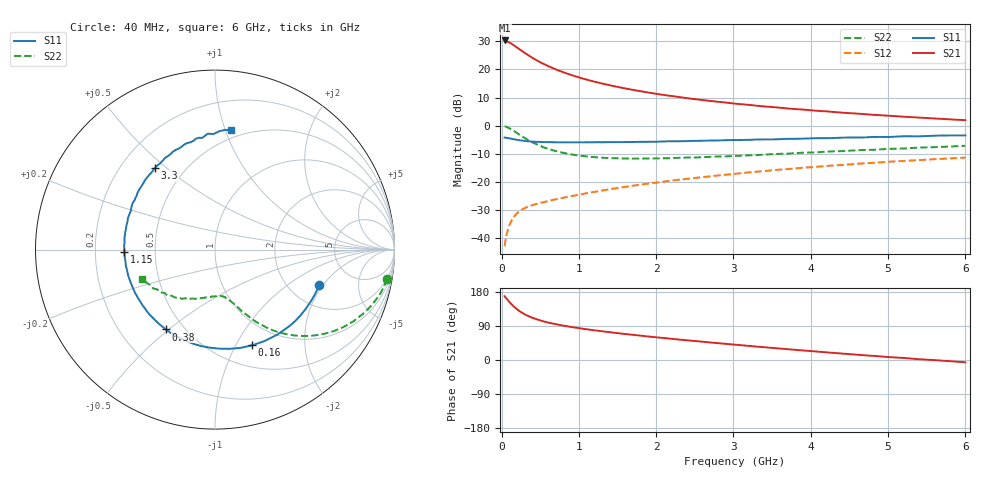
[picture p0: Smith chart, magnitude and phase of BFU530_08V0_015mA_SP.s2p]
! Filename:  P:\Prog\Test\Noise\ATS_data\Testdata_Net\03 Spar\BFU530_APG2013_40_A05_08p0V_015mA_SP_CM01_D.s2p
! Date/Time: Fri 26/Apr/2013 13:03:13
! BFU530_APG2013_40_A05_08p0V_1to25mA_SP_CM01_Bias6_R.s2p
! MDIF S-parameter v. bias file
! BFU530_APG2013_40_A05_08p0V_1to25mA_SP_CM01
! Date/time Wed Apr 24 16:58:28 2013
! VAR V_out= 8.0000
! VAR I_out= 14.9950
! VAR V_in= 0.8199
! VAR I_in= 0.1591
! Device data file deembeded for feedlines and parallel
! Original file: \03 Spar\BFU530_APG2013_40_A05_08p0V_015mA_SP_CM01_R.s2p
! Feed-files: PR047V01_250413_Feed1.s2p, PR047V01_250413_Feed2.s2p
! Parallel-file: PR047V01_250413_Par.s2p
# MHz S MA R 50
!  Freq-MHz  S11-mag  S11-arg  S21-mag  S21-arg  S12-mag  S12-arg  S22-mag  S22-arg
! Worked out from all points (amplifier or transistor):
!   98 points, 40 MHz to 6 GHz, reference 50 ohm
!   highest |S21| = 30.3 dB at 40 MHz (marker M1)
!   |S21| within 3 dB of that: start of sweep to 226.2 MHz
!   unconditionally stable (mu >= 1): 1.53 GHz to 3.802 GHz
!   at 300 MHz: K = 0.39, MSG = 27.6 dB, |S12| = -29.4 dB
!   at 1.6 GHz: K = 1.01, MAG = 16.8 dB, |S12| = -21.8 dB
!   at 6 GHz: K = 0.87, MSG = 6.7 dB, |S12| = -11.4 dB
!   S11 on the Smith chart (normalised r, x): 40 MHz: 2.89, -1.84; 160 MHz: 0.74, -1.17; 380 MHz: 0.40, -0.49; 1.15 GHz: 0.33, -0.01; 3.3 GHz: 0.34, +0.46; 6 GHz: 0.44, +1.05
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40  0.6132 -18.9  32.73 168.4  0.007166 82.0  0.9714 -9.7
50  0.6104 -23.6  32.58 165.4  0.008843 79.9  0.9648 -12.2
100  0.5949 -45.7  30.09 153.6  0.01661 71.2  0.8991 -23.4
120  0.5872 -54.0  29.08 149.0  0.01925 68.1  0.8681 -27.4
160  0.572 -68.8  26.75 141.0  0.02385 62.8  0.8031 -34.4
220  0.5524 -87.7  23.5 130.9  0.02904 57.2  0.708 -42.8
260  0.5432 -98.1  21.48 125.4  0.03172 54.5  0.6519 -47.2
320  0.5309 -111.1  18.88 118.5  0.03497 51.8  0.5806 -52.5
380  0.5225 -121.6  16.69 113.0  0.0376 50.1  0.5217 -56.5
440  0.5161 -130.2  14.92 108.5  0.03995 49.3  0.4748 -59.5
500  0.5121 -137.4  13.44 104.6  0.04212 48.9  0.4369 -62.1
650  0.5065 -151.5  10.73 96.7  0.04714 49.2  0.3695 -66.8
850  0.5045 -164.4  8.403 89.0  0.0538 50.5  0.3167 -71.1
1050  0.5042 -174.6  6.888 82.6  0.06076 52.0  0.2883 -74.9
1150  0.5048 -178.6  6.312 79.8  0.06437 52.5  0.2784 -76.5
1600  0.5102 165.7  4.581 68.5  0.08127 54.0  0.26 -84.2
2050  0.5199 154.2  3.589 59.0  0.09865 53.9  0.2615 -92.1
3100  0.5556 130.2  2.404 39.0  0.1424 50.6  0.2924 -110.8
3300  0.565 126.2  2.262 35.4  0.1513 49.5  0.299 -114.2
4100  0.5971 111.3  1.828 21.9  0.1863 44.4  0.3362 -127.7
5200  0.6472 93.5  1.442 5.4  0.2354 35.9  0.3914 -145.5
6000  0.6699 82.2  1.249 -6.0  0.2695 28.7  0.4371 -157.8
